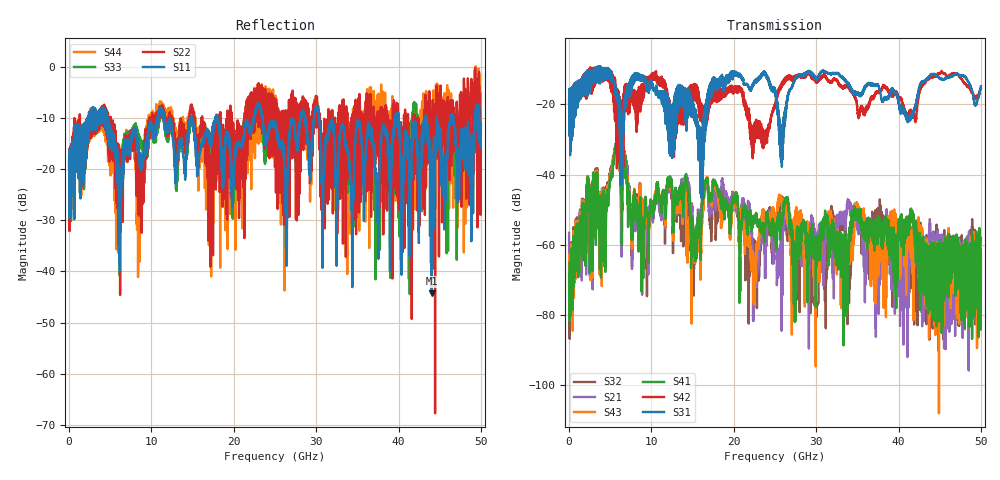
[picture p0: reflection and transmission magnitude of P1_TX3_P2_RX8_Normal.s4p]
!Keysight Technologies,N5225B,MY57041031,A.13.20.10
!Date: Friday, May 31, 2019 11:40:18
!Correction: S11(Full 4 Port(1,2,3,4))
!S12(Full 4 Port(1,2,3,4))
!S13(Full 4 Port(1,2,3,4))
!S14(Full 4 Port(1,2,3,4))
!S21(Full 4 Port(1,2,3,4))
!S22(Full 4 Port(1,2,3,4))
!S23(Full 4 Port(1,2,3,4))
!S24(Full 4 Port(1,2,3,4))
!S31(Full 4 Port(1,2,3,4))
!S32(Full 4 Port(1,2,3,4))
!S33(Full 4 Port(1,2,3,4))
!S34(Full 4 Port(1,2,3,4))
!S41(Full 4 Port(1,2,3,4))
!S42(Full 4 Port(1,2,3,4))
!S43(Full 4 Port(1,2,3,4))
!S44(Full 4 Port(1,2,3,4))
!S4P File: Measurements: <S11,S12,S13,S14>,
!<S21,S22,S23,S24>,
!<S31,S32,S33,S34>,
!<S41,S42,S43,S44>:
# Hz S  dB  R 50.0
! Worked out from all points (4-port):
!   5000 points, 10 MHz to 50 GHz, reference 50 ohm
!   strongest paths, dB at 10 MHz, 12.51 GHz, 25.01 GHz, 37.51 GHz, 50 GHz:
!     S31: -19.4, -27.1, -15.7, -14.5, -14.9
!     S42: -19.6, -21.6, -19.9, -16.6, -15.6
!     S41: -68.3, -43.3, -57.1, -53.3, -62.9
!     S43: -62.8, -44.0, -51.3, -68.9, -65.8
!     S21: -56.6, -45.7, -57.0, -72.6, -74.7
!     S32: -64.7, -46.9, -60.6, -50.5, -65.0
!   lowest |S11| = -44.3 dB at 44.03 GHz (marker M1), VSWR 1.01, Z = 49.8 + j0.591 ohm
!   |S11| at or under -10 dB: 4.66 GHz to 10.77 GHz (6.106 GHz wide, 79.2 % of centre); 23.49 GHz to 28.08 GHz (4.584 GHz wide, 17.8 % of centre); 30.37 GHz to 39.61 GHz (9.239 GHz wide, 26.4 % of centre)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
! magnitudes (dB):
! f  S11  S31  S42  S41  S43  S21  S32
! 10 MHz  -19.5  -19.4  -19.6  -68.3  -62.8  -56.6  -64.7
! 5.77 GHz  -20.0  -17.5  -20.0  -32.1  -31.8  -31.7  -31.4
! 9.44 GHz  -14.9  -14.9  -13.8  -51.5  -53.5  -59.0  -64.8
! 16.65 GHz  -12.9  -22.5  -25.3  -41.3  -41.4  -41.9  -42.1
! 22.58 GHz  -8.8  -13.2  -25.1  -51.7  -66.1  -65.9  -63.5
! 44.03 GHz  -44.3  -11.4  -12.4  -63.5  -74.2  -63.7  -66.1
! 50 GHz  -12.4  -14.9  -15.6  -62.9  -65.8  -74.7  -65.0
